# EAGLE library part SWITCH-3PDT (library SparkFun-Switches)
3-Pole, Double-Throw (3PDT) Switch Three-pole, double-throw stomp switch. Drawn as three separate gates for schematic clarity. SparkFun Products Used in SparkFun Proto Pedal (PRT-13124)
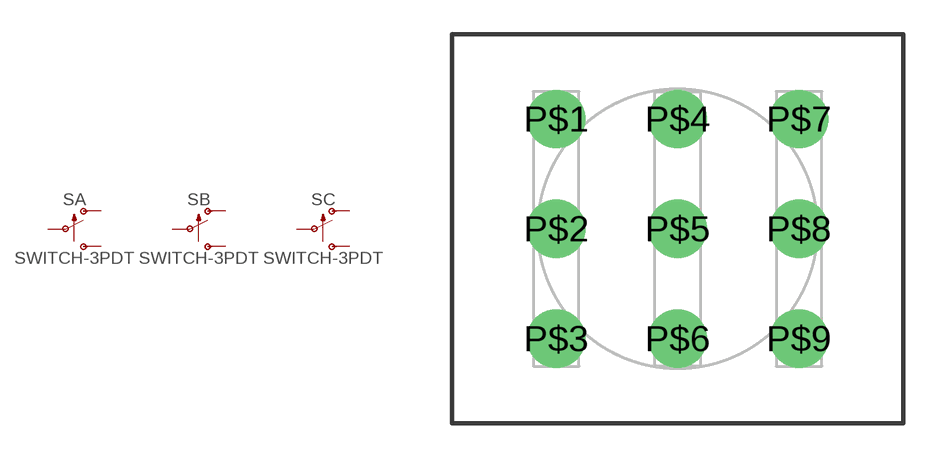
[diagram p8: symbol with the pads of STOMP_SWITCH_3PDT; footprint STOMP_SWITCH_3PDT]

Designator prefix S; gates A=SW_SPDT_POL B=SW_SPDT_POL C=SW_SPDT_POL

## SWITCH-3PDT-PTH-STOMP (PROD_ID: SWCH-13197)  [STOMP_SWITCH_3PDT]
P$1  A:O  pas
P$2  A:P  pas
P$3  A:S  pas
P$4  B:O  pas
P$5  B:P  pas
P$6  B:S  pas
P$7  C:O  pas
P$8  C:P  pas
P$9  C:S  pas

## Footprint STOMP_SWITCH_3PDT (pad centres in mm)
3-Pole, Double-Throw (3PDT) Stomp Switch Three-pole, double-throw stomp switch. Drawn as three separate gates for schematic clarity. Datasheet
drill 1.2 pad 2.54: P$1 -5.3,4.8; P$2 -5.3,0; P$3 -5.3,-4.8; P$4 0,4.8; P$5 0,0; P$6 0,-4.8; P$7 5.3,4.8; P$8 5.3,0; P$9 5.3,-4.8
